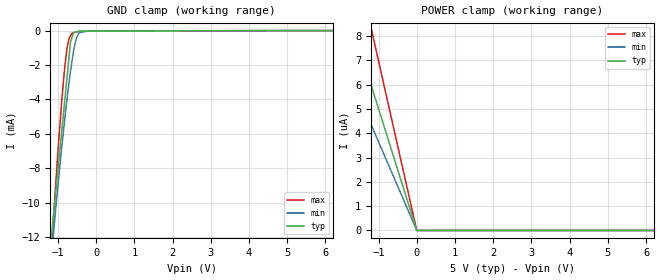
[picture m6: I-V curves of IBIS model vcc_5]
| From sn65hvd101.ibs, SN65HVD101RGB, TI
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|   vcc_5 Model
[Model]   vcc_5
Model_type   Input
Vinl = 0.8
Vinh = 2.0
|   typ   min   max
|   (nom PVT)   (fast PVT)   (slow PVT)
C_comp   8.085e-13   7.971e-13   8.143e-13
| Where nom  PVT is Nominal Process, 5V, 45C
|   Fast PVT is Strong Process,  5.5V, -20C
|   Slow PVT is Weak Process,   4.5V, 125C
[Voltage Range]   5   4.5   5.5
|Junction Temperature
[Temperature Range]   45   125   -20
[Power Clamp Reference]   5   4.5   5.5
[GND Clamp Reference]   0   0   0
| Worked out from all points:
|   GND clamp passes 1 mA (typ) near -0.69 V on its own axis
[GND Clamp]
|   Voltage   I(typ)   I(min)   I(max)
-5V       -180.4mA   -153.1mA   -213.8mA
-1.243V   -14.37mA   -15.02mA   -15.29mA
-1.14V    -11.3mA    -12.43mA   -11.69mA
-1.105V   -10.52mA   -11.56mA   -10.49mA
-907.5mV  -6.029mA   -6.949mA   -4.309mA
-819.5mV  -4.033mA   -5.122mA   -2.089mA
-759mV    -2.661mA   -3.937mA   -981.5uA
-670mV    -641.9uA   -2.345mA   -302.9uA
-585mV    -112.9uA   -1.113mA   -124.8uA
-445.5mV  -34.16uA   -122.5uA   -42.14uA
-202.5mV  -26.53uA   -17.32uA   -39.99uA
10V       0A         0A         0A
[POWER Clamp]
|   Voltage   I(typ)   I(min)   I(max)
-5V       25.06uA    18.24uA    34.88uA
-2.268V   11.37uA    8.272uA    15.82uA
-1.375V   6.891uA    5.015uA    9.592uA
-1.14V    5.713uA    4.158uA    7.952uA
-84.44fV  0A         0A         0A
10V       0A         0A         0A
